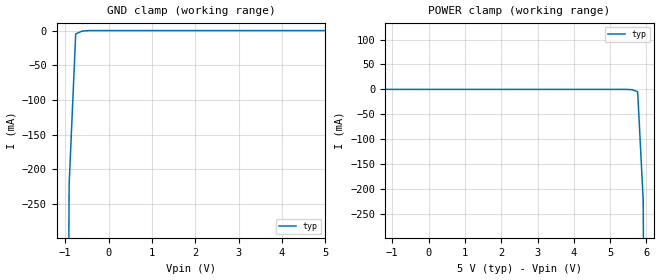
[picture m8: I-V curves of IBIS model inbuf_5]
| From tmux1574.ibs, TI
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| inbuf_5
[Model]   inbuf_5
Model_type   Input
Vinl = 0.45
Vinh = 1.2
|   typ   min   max
C_comp   2.533030e-12   NA   NA
[Voltage Range]   5   NA   NA
[Temperature Range]   27   NA   NA
[Power Clamp Reference]   5   NA   NA
[GND Clamp Reference]   0   NA   NA
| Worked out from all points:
|   GND clamp passes 1 mA (typ) near -0.62 V on its own axis
|   POWER clamp passes 1 mA (typ) near -3.65 V on its own axis
[GND Clamp]
|   Voltage   I(typ)   I(min)   I(max)
-10V      -181.4A    NA         NA
-1.061V   -2.062A    NA         NA
-909.1mV  -221.5mA   NA         NA
-757.6mV  -4.809mA   NA         NA
-606.1mV  -650.5uA   NA         NA
-454.5mV  -36.69uA   NA         NA
5V        833.5nA    NA         NA
[POWER Clamp]
|   Voltage   I(typ)   I(min)   I(max)
-5V       122.7mA    NA         NA
-3.939V   21.18mA    NA         NA
-3.788V   8.414mA    NA         NA
-3.636V   511.7uA    NA         NA
5.606V    -650.5uA   NA         NA
5.758V    -4.809mA   NA         NA
5.909V    -221.5mA   NA         NA
6.061V    -2.062A    NA         NA
10V       -80.19A    NA         NA
